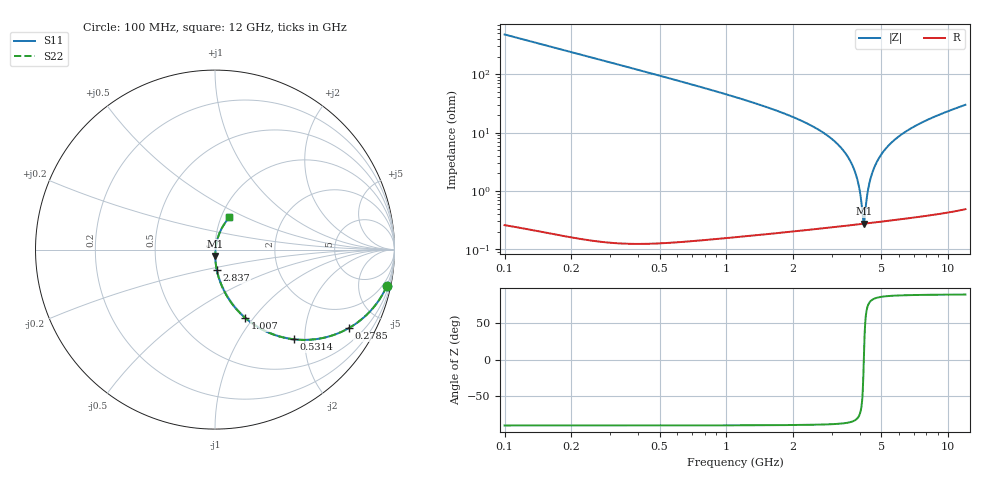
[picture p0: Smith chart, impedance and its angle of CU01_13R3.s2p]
! S-parameter model data by Modelithics Inc. support@modelithics.com 813-866-6335 Tampa FL USA
! S-Parameter data specifications:
! Substrate: 20-mil Rogers, substrate thickness, H=0.508mm, Dielectric constant, Er=3.75
! PCB Mounting Pad Footprint: Pad width, PadW=0.35mm , Pad length, PadL=0.30mm , Pad gap, PadG (edge-to-edge)=0.25mm , Reference planes=0.85mm apart
! Created Wed May 09 13:18:47 2018
# hz S ma R 50
! 2 Port Network Data from SP1.SP block
! freq  magS11  angS11  magS21  angS21  magS12  angS12  magS22  angS22
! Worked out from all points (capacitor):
!   801 points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, 100 MHz to 12 GHz, reference 50 ohm
!   read as one part in series: C = 3.32 pF near 159.5 MHz
!   lowest |Z| = 275 mohm at 4.176 GHz (marker M1)
!   series resonance near 4.177 GHz, so ESL is about 440 pH
!   S11 on the Smith chart (normalised r, x): 100 MHz: 0.99, -9.50; 278.5 MHz: 0.99, -3.40; 531.4 MHz: 0.99, -1.77; 1.007 GHz: 0.99, -0.91; 2.837 GHz: 0.99, -0.23; 12 GHz: 1.10, +0.41
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1e8  0.9788 -11.9  0.2045 78.1  0.2045 78.1  0.9788 -11.9
2.785e8  0.8635 -30.5  0.5037 59.4  0.5037 59.4  0.8635 -30.5
5.31375e8  0.6648 -48.8  0.7461 41.2  0.7461 41.2  0.6648 -48.8
7.39625e8  0.5346 -58.3  0.8439 31.6  0.8439 31.6  0.5346 -58.3
1.007375e9  0.4145 -66.3  0.9086 23.5  0.9086 23.5  0.4145 -66.3
2.09325e9  0.1853 -80.7  0.9806 8.7  0.9806 8.7  0.1853 -80.7
2.837e9  0.1138 -85.0  0.9912 3.8  0.9912 3.8  0.1138 -85.0
4.071625e9  0.03974 -87.7  0.9965 -1.6  0.9965 -1.6  0.03974 -87.7
4.17575e9  0.03482 -87.5  0.9966 -2.0  0.9966 -2.0  0.03482 -87.5
4.65175e9  0.01409 -82.0  0.997 -3.6  0.997 -3.6  0.01409 -82.0
4.77075e9  0.009379 -76.2  0.997 -4.0  0.997 -4.0  0.009379 -76.2
4.94925e9  0.003453 -36.8  0.997 -4.6  0.997 -4.6  0.003453 -36.8
4.993875e9  0.002935 -6.9  0.997 -4.8  0.997 -4.8  0.002935 -6.9
5.053375e9  0.003665 31.5  0.997 -4.9  0.997 -4.9  0.003665 31.5
5.231875e9  0.009379 65.9  0.9969 -5.5  0.9969 -5.5  0.009379 65.9
5.3955e9  0.01516 72.5  0.9968 -6.0  0.9968 -6.0  0.01516 72.5
5.678125e9  0.025 76.0  0.9965 -6.8  0.9965 -6.8  0.025 76.0
6.05e9  0.03742 77.2  0.996 -7.9  0.996 -7.9  0.03742 77.2
6.868125e9  0.06292 76.8  0.9945 -10.1  0.9945 -10.1  0.06292 76.8
8.04325e9  0.09644 74.6  0.9915 -13.2  0.9915 -13.2  0.09644 74.6
1.002162e10  0.1481 70.3  0.9847 -18.1  0.9847 -18.1  0.1481 70.3
1.2e10  0.1971 65.9  0.9755 -22.8  0.9755 -22.8  0.1971 65.9
